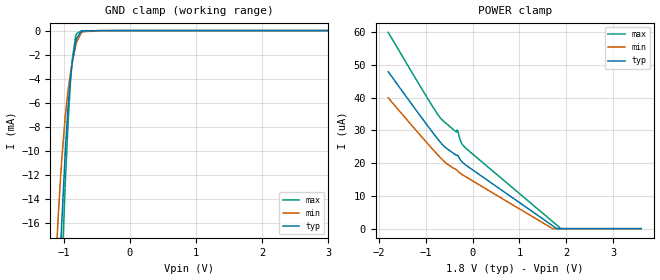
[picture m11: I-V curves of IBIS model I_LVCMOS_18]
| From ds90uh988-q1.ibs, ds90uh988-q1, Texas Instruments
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[Model]   I_LVCMOS_18
Model_type   Input
Vinl = 0.63
Vinh = 1.17
|   typ   min   max
C_comp   0.697pF   0.730pF   0.666pF
[Voltage Range]   1.8   1.71   1.89
[Temperature Range]   27   105   -40
[Power Clamp Reference]   1.8   1.71   1.89
[GND Clamp Reference]   0   0   0
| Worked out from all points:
|   GND clamp passes 1 mA (typ) near -0.82 V on its own axis
[GND Clamp]
|   Voltage   I(typ)   I(min)   I(max)
-1.8V     -133.4mA   -111.8mA   -151.5mA
-1.147V   -31.86mA   -22.51mA   -38.55mA
-1.082V   -22.95mA   -15.61mA   -28.27mA
-1.033V   -16.75mA   -11.25mA   -20.95mA
-1.028V   -16.09mA   -10.82mA   -20.17mA
-973.8mV  -10.12mA   -7.141mA   -12.77mA
-936mV    -6.72mA    -5.199mA   -8.223mA
-892.8mV  -3.83mA    -3.452mA   -4.055mA
-871.2mV  -2.769mA   -2.724mA   -2.53mA
-817.2mV  -982.2uA   -1.276mA   -474.4uA
-730.8mV  -68.67uA   -178.6uA   -22.21uA
3.6V      0A         0A         0A
[POWER Clamp]
|   Voltage   I(typ)   I(min)   I(max)
-1.8V     47.91uA    39.97uA    59.93uA
-774mV    27.93uA    23.03uA    35.55uA
-590.4mV  24.94uA    20.34uA    32.46uA
-347.4mV  22.42uA    18.03uA    29.53uA
-325.8mV  22.45uA    17.72uA    30.04uA
-309.6mV  22.25uA    17.49uA    29.6uA
-261mV    21.05uA    16.91uA    27.01uA
-207mV    20.16uA    16.39uA    25.52uA
1.705V    950nA      43.82nA    2.234uA
1.796V    33.38nA    0A         1.123uA
1.888V    0A         0A         8.941nA
3.6V      0A         0A         0A
